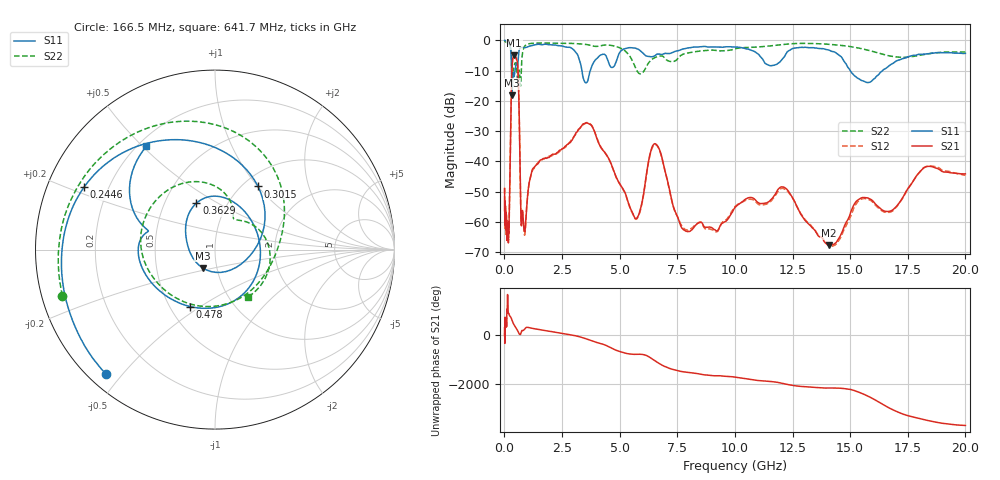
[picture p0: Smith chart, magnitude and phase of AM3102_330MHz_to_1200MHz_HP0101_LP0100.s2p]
! Date/Time: Tue, Sep 11, 2018 5:13 PM
! Network Analyzer: Agilent Technologies E8362B Rev: A.07.50.63
! Sweep from 0.010 to 20.000 GHz, 1601 Points, Sweep Type: LOG
! Power Supply: 4.949 V, 0.001 A
# Hz S DB R 50
!freq MagS11 AngS11 MagS21 AngS21 MagS12 AngS12 MagS22 AngS22
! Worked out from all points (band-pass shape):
!   1601 points, 10 MHz to 20 GHz, reference 50 ohm
!   highest |S21| = -4.97 dB at 424.4 MHz (marker M1); lowest = -67.7 dB at 14.07 GHz (marker M2)
!   |S21| within 3 dB of the highest: 337.4 MHz to 574 MHz (236.6 MHz wide, 51.9 % of centre)
!   lowest |S11| = -18.2 dB at 333.1 MHz (marker M3), VSWR 1.28, Z = 42.7 - j8.84 ohm
!   |S11| at or under -10 dB: 309.5 MHz to 460.6 MHz (151.1 MHz wide, 39.3 % of centre); 3.363 GHz to 3.726 GHz (362.7 MHz wide, 10.2 % of centre); 15.01 GHz to 16.4 GHz (1.399 GHz wide, 8.91 % of centre)
!   |S22| runs from -15.2 to -0.2 dB; largest |S21 - S12| = 0.0091
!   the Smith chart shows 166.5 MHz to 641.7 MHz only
!   S11 on the Smith chart (normalised r, x): 166.5 MHz: 0.05, -0.45; 244.6 MHz: 0.11, +0.23; 301.5 MHz: 1.17, +1.00; 362.9 MHz: 0.72, +0.40; 478 MHz: 0.63, -0.45; 641.7 MHz: 0.23, +0.51
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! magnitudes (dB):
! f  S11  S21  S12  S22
! 10 MHz  0.0  -48.9  -48.8  -0.2
! 35.55 MHz  0.0  -59.7  -59.6  -0.4
! 126.4 MHz  -0.4  -64.3  -63.0  -0.8
! 166.5 MHz  -0.7  -65.5  -64.3  -1.0
! 244.6 MHz  -1.9  -43.6  -43.6  -1.9
! 301.5 MHz  -7.4  -17.3  -17.3  -4.3
! 333.1 MHz  -18.2  -8.6  -8.6  -8.5
! 362.9 MHz  -11.1  -6.1  -6.2  -10.4
! 424.4 MHz  -11.9  -5.0  -5.0  -8.4
! 447.2 MHz  -10.7  -5.1  -5.1  -7.7
! 478 MHz  -9.2  -5.3  -5.4  -7.4
! 641.7 MHz  -3.2  -24.1  -24.2  -9.9
! 726 MHz  -2.3  -60.3  -60.3  -11.7
! 873.8 MHz  -2.4  -63.0  -64.2  -2.0
! 1.59 GHz  -1.4  -39.5  -39.5  -0.9
! 3.668 GHz  -11.6  -27.6  -27.3  -1.5
! 5.652 GHz  -2.5  -58.6  -58.7  -8.4
! 6.58 GHz  -4.8  -34.3  -34.5  -5.5
! 7.845 GHz  -2.7  -62.9  -62.6  -4.3
! 12.09 GHz  -5.9  -48.5  -48.9  -1.4
! 14.07 GHz  -3.2  -67.7  -67.5  -1.3
! 20 GHz  -4.3  -44.1  -44.6  -3.8
